| TI TMS320DM355 ZCE IBIS MODEL
[IBIS ver] 3.2
[File_name] sprm271a.ibs
[File Rev]   1.30
[Date]   October 24, 2007
[Source]   TIH DSP design
[Notes]   This data is based on 3/14/06 package substrate.
   Voltage of IO is VDDS +5%, -10%.
   EM_A08/10/11 are changed from PD to PU. [1.10]
   Updated pin file   [1.20]
   Updated some of IO model   [1.20]
   ADDED DDR pins support   [1.30]
[Disclaimer]   This information is for modeling purpose only, and is
   not guaranteed.
   The information is subject to change without notice.
[Copyright]   Property of Texas Instruments Incorporated. Unauthorized
   reproduction and/or distribution is strictly prohibited. This
   product is protected under copyright law and trade secret law
   as an unpublished work. Copyright (C) 2006, Texas Instruments
   Incorporated, all rights reserved. These commodities are under
   the U.S. Government distribution license control. As such,
   they are not to be re-exported without the prior approval of
   the U.S. Department of Commerce.
| Component   TMS320DM355 ZCE
[Component]   TMS320DM355ZCE
[Manufacturer] Texas Instruments
[Package]
| variable   typ   min   max
R_pkg   2.34767E-001  1.09280E-001  3.31800E-001
L_pkg   3.54436E-009  1.69380E-009  6.02860E-009
C_pkg   7.29148E-013  4.32190E-013  1.42590E-012
[Pin]signal_name   model_name   R_pin   L_pin   C_pin
G3   EXTCLK   BC3325DTHYPD   2.24E-01   3.68E-09   6.78E-13
C3   YOUT7   BC3325DTHYPD   1.96E-01   3.10E-09   4.95E-13
B3   YOUT4   BC3325DTHYPD   2.78E-01   4.88E-09   7.97E-13
B4   YOUT5   BC3325DTHYPD   3.26E-01   6.03E-09   9.32E-13
A4   YOUT6   BC3325DTHYPD   2.71E-01   4.71E-09   7.32E-13
B2   YOUT3   BC3325DTHYPD   2.52E-01   4.56E-09   8.47E-13
A3   YOUT2   BC3325DTHYPD   2.98E-01   5.52E-09   8.15E-13
A2   YOUT1   BC3325DTHYPD   2.79E-01   5.46E-09   8.87E-13
B1   YOUT0   BC3325DTHYPD   2.68E-01   4.80E-09   8.71E-13
D2   COUT6   BC3325DTHYPD   2.51E-01   3.93E-09   7.90E-13
L5   YIN7   BC3350CTHYPD   1.39E-01   2.19E-09   7.55E-13
N3   CIN7   BC3350CTHYPD   2.40E-01   3.18E-09   9.57E-13
M3   CIN5   BC3350CTHYPD   2.64E-01   3.86E-09   7.08E-13
M4   YIN6   BC3350CTHYPD   2.64E-01   3.41E-09   1.04E-12
P5   YIN0   BC3350CTHYPD   2.60E-01   3.76E-09   1.22E-12
M5   YIN5   BC3350CTHYPD   2.98E-01   4.46E-09   1.34E-12
R3   YIN3   BC3350CTHYPD   2.77E-01   4.03E-09   8.58E-13
P4   YIN2   BC3350CTHYPD   2.01E-01   2.55E-09   8.40E-13
P3   YIN4   BC3350CTHYPD   2.67E-01   3.81E-09   9.00E-13
P2   YIN1   BC3350CTHYPD   2.97E-01   4.54E-09   1.18E-12
H5   LCD_OE   BC3325DTHYPD   2.32E-01   3.10E-09   6.60E-13
H4   FIELD   BC3325DTHYPD   1.86E-01   2.46E-09   5.37E-13
G5   VSYNC   BC3325DTHYPD   1.82E-01   2.38E-09   5.53E-13
F5   HSYNC   BC3325DTHYPD   2.28E-01   3.17E-09   7.08E-13
J9   VSSA_PLL2   GND   NA   NA   NA
H12   VSSA_PLL1   GND   NA   NA   NA
R11   VSSA_DLL   GND   NA   NA   NA
U10   VREFSSTL   POWER   NA   NA   NA
R10   VDDAHV33_DLL   POWER   NA   NA   NA
H9   VDDA_PLL2   POWER   NA   NA   NA
E8   EMU0   BC3325DTHYPU   2.57E-01   3.30E-09   1.02E-12
G12   VDDA_PLL1   POWER   NA   NA   NA
D11   RESETN   IC33THYPU   2.56E-01   3.26E-09   8.09E-13
C11   CLKOUT3   BC3350CTHYPD   1.96E-01   2.57E-09   7.51E-13
H3   VCLK   BC3325DSHYPD   1.87E-01   2.45E-09   5.52E-13
R17   UART1_TXD   BC3350ASHYPD   1.86E-01   2.72E-09   6.26E-13
R15   UART1_RXD   BC3350ASHYPD   2.02E-01   2.70E-09   9.58E-13
U18   UART0_RXD   IC33SHYPD   2.32E-01   3.57E-09   7.82E-13
T18   UART0_TXD   OC3350AS   2.16E-01   3.33E-09   6.87E-13
D8   TMS   IC33THYPU   2.63E-01   3.30E-09   7.20E-13
D9   TDI   IC33THYPU   2.81E-01   3.50E-09   6.13E-13
E9   TDO   OC3325DT   2.44E-01   2.99E-09   7.89E-13
E10   TCK   IC33THYPU   3.10E-01   4.93E-09   8.89E-13
E12   SPI1_SDO   BC3350CTHYPD   2.02E-01   2.75E-09   6.28E-13
A13   SPI1_SDI   BC3350CTHYPD   2.58E-01   4.15E-09   5.96E-13
C13   SPI1_SCLK   BC3350CTHYPD   2.04E-01   2.76E-09   7.60E-13
E13   SPI1_SDENA0   BC3350CTHYPD   2.79E-01   3.93E-09   8.91E-13
D14   MMCSD0_DATA1   BC3350CTHYPD   2.61E-01   3.43E-09   8.23E-13
B11   SPI0_SDO   BC3350CTHYPD   2.51E-01   3.72E-09   6.74E-13
D12   CLKOUT1   BC3350CTHYPD   2.25E-01   3.01E-09   6.78E-13
A12   SPI0_SDI   BC3350CTHYPD   2.34E-01   3.88E-09   6.07E-13
B12   SPI0_SDENA0   BC3350CTHYPD   2.70E-01   3.75E-09   6.15E-13
C12   SPI0_SCLK   BC3350CTHYPD   2.21E-01   3.17E-09   6.93E-13
E14   GIO001   BC3365ATHYPD   2.35E-01   3.09E-09   1.05E-12
J3   CIN0   BC3350CTHYPD   2.70E-01   4.04E-09   8.54E-13
B16   MMCSD1_DATA3   BC3350CTHYPD   2.33E-01   3.81E-09   6.66E-13
A15   MMCSD0_CLK   BC3350CTHYPD   2.67E-01   4.46E-09   6.01E-13
C16   GIO000   BC3365ATHYPD   2.73E-01   4.09E-09   8.36E-13
A16   MMCSD1_DATA2   BC3350CTHYPD   2.48E-01   4.17E-09   5.81E-13
B15   MMCSD1_DATA1   BC3350CTHYPD   2.44E-01   3.74E-09   6.10E-13
A17   MMCSD1_CMD   BC3350CTHYPD   2.74E-01   4.58E-09   6.24E-13
A18   MMCSD1_DATA0   BC3350CTHYPD   2.77E-01   5.82E-09   7.92E-13
C14   MMCSD0_CMD   BC3350CTHYPD   2.27E-01   3.65E-09   7.84E-13
C15   MMCSD1_CLK   BC3350CTHYPD   2.06E-01   2.68E-09   7.39E-13
B18   GIO006   BC3365ATHYPD   2.87E-01   4.64E-09   6.99E-13
A14   MMCSD0_DATA3   BC3350CTHYPD   2.62E-01   4.19E-09   5.94E-13
B13   MMCSD0_DATA2   BC3350CTHYPD   2.56E-01   3.91E-09   6.43E-13
B14   MMCSD0_DATA0   BC3350CTHYPD   2.30E-01   3.51E-09   9.89E-13
E11   RTCK   OC3325DT   2.48E-01   3.31E-09   6.96E-13
C9   TRSTN   IC33THYPD   2.04E-01   2.63E-09   4.65E-13
T3   PCLK   BC3350CTHYPD   1.22E-01   2.38E-09   8.68E-13
E16   ASP1_FSX   BC3350BSHYPD   1.82E-01   2.59E-09   1.05E-12
F17   ASP0_CLKR   BC3350BSHYPD   2.24E-01   2.88E-09   7.42E-13
D17   ASP1_CLKS   IC33SHYPD   2.03E-01   3.10E-09   8.02E-13
E17   ASP1_FSR   BC3350BSHYPD   2.46E-01   3.84E-09   7.20E-13
F16   ASP0_FSR   BC3350BSHYPD   1.79E-01   2.30E-09   8.28E-13
D19   ASP1_CLKX   BC3350BSHYPD   2.53E-01   4.18E-09   5.69E-13
C18   ASP1_DX   BC3350BSHYPD   2.24E-01   3.75E-09   6.87E-13
D18   ASP1_CLKR   BC3350BSHYPD   2.11E-01   3.33E-09   5.56E-13
C19   ASP1_DR   BC3350BSHYPD   2.56E-01   4.43E-09   6.92E-13
G17   ASP0_FSX   BC3350BSHYPD   1.71E-01   2.28E-09   5.88E-13
E18   ASP0_DR   BC3350BSHYPD   2.30E-01   3.86E-09   6.62E-13
H15   ASP0_DX   BC3350BSHYPD   1.79E-01   2.34E-09   6.24E-13
G19   EM_CE1   BC3350CSHYPD   2.40E-01   4.05E-09   5.45E-13
F18   ASP0_CLKX   BC3350BSHYPD   2.16E-01   3.38E-09   6.61E-13
R13   I2C_SDA   BC3350BSHYPD   3.22E-01   4.17E-09   1.13E-12
R14   I2C_SCL   BC3350BSHYPD   2.43E-01   3.14E-09   1.02E-12
E4   COUT2   BC3325DTHYPD   2.20E-01   3.31E-09   6.32E-13
C17   GIO007   BC3350CTHYPD   2.25E-01   3.48E-09   7.55E-13
D15   GIO005   BC3365ATHYPD   2.11E-01   2.63E-09   8.41E-13
B17   GIO004   BC3365ATHYPD   2.72E-01   4.04E-09   6.65E-13
G15   GIO003   BC3365ATHYPD   2.63E-01   3.75E-09   1.12E-12
F15   GIO002   BC3365ATHYPD   3.18E-01   4.17E-09   1.13E-12
E7   EMU1   BC3325DTHYPU   2.77E-01   3.78E-09   9.43E-13
J15   EM_WE   BC3350CSHYPD   1.83E-01   2.47E-09   6.58E-13
H16   EM_ADV   BC3350CSHYPD   1.69E-01   2.18E-09   6.65E-13
F19   EM_OE   BC3350CSHYPD   2.53E-01   4.47E-09   6.15E-13
G18   EM_WAIT   BC3350CSHYPU   2.11E-01   3.12E-09   6.97E-13
E19   EM_CLK   BC3350CSHYPD   2.53E-01   4.48E-09   7.16E-13
H18   EM_D00   BC3350CSHYPD   2.09E-01   3.17E-09   5.66E-13
J16   EM_CE0   BC3350CSHYPD   1.88E-01   2.45E-09   7.90E-13
K18   EM_D09   BC3350CSHYPD   2.09E-01   3.14E-09   5.13E-13
L17   EM_D11   BC3350CSHYPD   1.70E-01   2.32E-09   6.00E-13
K19   EM_D07   BC3350CSHYPD   2.30E-01   3.76E-09   4.32E-13
L16   EM_D08   BC3350CSHYPD   1.80E-01   2.42E-09   5.40E-13
K17   EM_D06   BC3350CSHYPD   1.74E-01   2.35E-09   6.18E-13
L19   EM_D10   BC3350CSHYPD   2.30E-01   3.75E-09   4.84E-13
J19   EM_D05   BC3350CSHYPD   2.32E-01   3.80E-09   5.15E-13
J18   EM_D03   BC3350CSHYPD   2.09E-01   3.10E-09   5.35E-13
L15   EM_D04   BC3350CSHYPD   1.86E-01   2.61E-09   7.42E-13
H19   EM_D02   BC3350CSHYPD   2.33E-01   3.84E-09   5.25E-13
J17   EM_D01   BC3350CSHYPD   1.82E-01   2.38E-09   5.78E-13
M18   EM_D15   BC3350CSHYPD   2.01E-01   3.08E-09   7.29E-13
M19   EM_D14   BC3350CSHYPD   2.37E-01   3.99E-09   5.53E-13
M15   EM_D13   BC3350CSHYPD   1.88E-01   2.62E-09   6.90E-13
L18   EM_D12   BC3350CSHYPD   2.41E-01   3.76E-09   6.14E-13
P19   EM_BA1   BC3350CSHYPD   2.49E-01   4.15E-09   6.53E-13
N19   EM_BA0   BC3350CSHYPD   2.40E-01   4.22E-09   6.24E-13
M16   EM_A00   BC3350CSHYPD   1.96E-01   2.56E-09   8.14E-13
P17   EM_A09   BC3350CSHYPD   1.71E-01   2.45E-09   6.27E-13
R18   EM_A10   BC3350CSHYPU   2.32E-01   3.69E-09   6.83E-13
T19   EM_A08   BC3350CSHYPU   2.60E-01   4.63E-09   7.18E-13
P18   EM_A06   BC3350CSHYPD   2.26E-01   3.53E-09   7.06E-13
P16   EM_A07   BC3350CSHYPD   1.77E-01   2.36E-09   9.18E-13
P15   EM_A04   BC3350CSHYPD   1.87E-01   2.60E-09   9.81E-13
R19   EM_A05   BC3350CSHYPD   2.54E-01   4.40E-09   7.09E-13
N18   EM_A03   BC3350CSHYPD   2.21E-01   3.25E-09   6.71E-13
N15   EM_A02   BC3350CSHYPD   1.83E-01   2.49E-09   9.24E-13
N17   EM_A01   BC3350CSHYPD   2.28E-01   3.20E-09   7.44E-13
V19   EM_A13   BC3350CSHYPD   2.56E-01   4.94E-09   6.57E-13
U19   EM_A12   BC3350CSHYPD   2.70E-01   4.79E-09   6.54E-13
R16   EM_A11   BC3350CSHYPU   1.84E-01   2.61E-09   7.83E-13
C2   COUT7   BC3325DTHYPD   2.66E-01   4.58E-09   8.29E-13
D3   COUT4   BC3325DTHYPD   2.14E-01   3.45E-09   7.31E-13
C1   COUT5   BC3325DTHYPD   2.56E-01   4.23E-09   7.11E-13
E3   COUT3   BC3325DTHYPD   2.71E-01   4.04E-09   8.99E-13
F3   COUT1   BC3325DTHYPD   3.20E-01   5.25E-09   1.12E-12
F4   COUT0   BC3325DTHYPD   1.79E-01   2.48E-09   5.17E-13
A11   CLKOUT2   BC3350CTHYPD   2.34E-01   3.76E-09   5.69E-13
K5   CIN6   BC3350CTHYPD   2.85E-01   4.98E-09   1.14E-12
L4   CIN4   BC3350CTHYPD   1.30E-01   1.89E-09   5.85E-13
J4   CIN3   BC3350CTHYPD   2.78E-01   4.31E-09   9.42E-13
L3   CIN1   BC3350CTHYPD   2.57E-01   3.51E-09   7.66E-13
J5   CIN2   BC3350CTHYPD   2.52E-01   4.09E-09   9.26E-13
R5   CAM_WEN_FIELD   BC3350CTHYPD   2.80E-01   3.85E-09   1.03E-12
N5   CAM_HD   BC3350CTHYPD   3.32E-01   4.97E-09   1.43E-12
R4   CAM_VD   BC3350CTHYPD   2.67E-01   3.52E-09   9.37E-13
T8   DDR_CS   BCSSTL18TCSCGPBFZP33   2.60E-01   3.33E-09   9.15E-13
V12   DDR_DQS0   BCSSTL18TCSCGPBFZP33   2.28E-01   3.17E-09   5.83E-13
V15   DDR_DQS1   BCSSTL18TCSCGPBFZP33   2.47E-01   3.53E-09   5.24E-13
W15   DDR_DQ11   BCSSTL18TCSCGPBFZP33   2.65E-01   3.98E-09   4.84E-13
W16   DDR_DQ13   BCSSTL18TCSCGPBFZP33   2.71E-01   4.35E-09   5.28E-13
U11   DDR_DQ2   BCSSTL18TCSCGPBFZP33   2.31E-01   3.04E-09   6.83E-13
V11   DDR_DQ0   BCSSTL18TCSCGPBFZP33   2.29E-01   3.12E-09   6.24E-13
U15   DDR_DQM1   BCSSTL18TCSCGPBFZP33   1.95E-01   2.57E-09   6.49E-13
W14   DDR_DQ10   BCSSTL18TCSCGPBFZP33   2.38E-01   3.67E-09   6.26E-13
V14   DDR_DQ9   BCSSTL18TCSCGPBFZP33   2.12E-01   3.09E-09   6.33E-13
U13   DDR_DQ8   BCSSTL18TCSCGPBFZP33   2.55E-01   3.13E-09   7.02E-13
V13   DDR_DQ6   BCSSTL18TCSCGPBFZP33   2.09E-01   3.15E-09   6.82E-13
W13   DDR_DQ7   BCSSTL18TCSCGPBFZP33   2.63E-01   3.96E-09   6.05E-13
U12   DDR_DQ4   BCSSTL18TCSCGPBFZP33   2.32E-01   3.04E-09   6.87E-13
W12   DDR_DQ5   BCSSTL18TCSCGPBFZP33   2.34E-01   4.00E-09   6.69E-13
T11   DDR_DQ3   BCSSTL18TCSCGPBFZP33   1.09E-01   1.69E-09   7.03E-13
W11   DDR_DQ1   BCSSTL18TCSCGPBFZP33   2.52E-01   3.71E-09   5.81E-13
U16   DDR_DQ12   BCSSTL18TCSCGPBFZP33   2.10E-01   3.07E-09   7.26E-13
V9   DDR_CAS   BCSSTL18TCSCGPBFZP33   2.28E-01   3.16E-09   6.48E-13
W9   DDR_CLKP   BCSSTL18TCSCGPBFZP33   2.28E-01   3.32E-09   6.12E-13
W8   DDR_CLKN   BCSSTL18TCSCGPBFZP33   2.27E-01   3.47E-09   5.96E-13
U6   DDR_A13   BCSSTL18TCSCGPBFZP33   1.93E-01   2.59E-09   7.80E-13
V10   DDR_CKE   BCSSTL18TCSCGPBFZP33   2.11E-01   3.10E-09   6.55E-13
V8   DDR_BA2   BCSSTL18TCSCGPBFZP33   2.04E-01   3.00E-09   6.39E-13
U8   DDR_BA0   BCSSTL18TCSCGPBFZP33   2.45E-01   3.10E-09   7.55E-13
U7   DDR_BA1   BCSSTL18TCSCGPBFZP33   2.22E-01   2.98E-09   6.50E-13
W6   DDR_A9   BCSSTL18TCSCGPBFZP33   2.62E-01   4.13E-09   5.43E-13
W7   DDR_A11   BCSSTL18TCSCGPBFZP33   2.55E-01   4.01E-09   5.72E-13
V5   DDR_A7   BCSSTL18TCSCGPBFZP33   2.15E-01   3.31E-09   5.94E-13
W5   DDR_A8   BCSSTL18TCSCGPBFZP33   2.62E-01   4.00E-09   5.05E-13
V6   DDR_A10   BCSSTL18TCSCGPBFZP33   2.09E-01   3.14E-09   6.17E-13
U5   DDR_A6   BCSSTL18TCSCGPBFZP33   1.95E-01   2.56E-09   7.42E-13
W4   DDR_A5   BCSSTL18TCSCGPBFZP33   2.67E-01   4.23E-09   5.04E-13
V4   DDR_A4   BCSSTL18TCSCGPBFZP33   2.23E-01   3.46E-09   6.09E-13
W3   DDR_A3   BCSSTL18TCSCGPBFZP33   2.78E-01   4.36E-09   5.80E-13
W2   DDR_A2   BCSSTL18TCSCGPBFZP33   2.83E-01   4.51E-09   6.46E-13
V3   DDR_A1   BCSSTL18TCSCGPBFZP33   2.34E-01   3.38E-09   6.40E-13
V7   DDR_A12   BCSSTL18TCSCGPBFZP33   2.05E-01   3.13E-09   6.01E-13
V2   DDR_A0   BCSSTL18TCSCGPBFZP33   2.79E-01   4.39E-09   7.45E-13
V17   DDR_STRBEN_DEL   BCSSTL18TCSCGPBFZP33   2.41E-01   3.55E-09   6.91E-13
W18   DDR_STRBEN   BCSSTL18TCSCGPBFZP33   2.97E-01   4.73E-09   6.68E-13
V16   DDR_DQ14   BCSSTL18TCSCGPBFZP33   2.61E-01   3.71E-09   6.02E-13
T6   DDR_RAS   BCSSTL18TCSCGPBFZP33   2.24E-01   3.24E-09   1.02E-12
W10   DDR_WE   BCSSTL18TCSCGPBFZP33   2.45E-01   3.86E-09   6.36E-13
T12   DDR_DQM0   BCSSTL18TCSCGPBFZP33   1.95E-01   2.53E-09   7.28E-13
W17   DDR_DQ15   BCSSTL18TCSCGPBFZP33   2.59E-01   4.27E-09   6.01E-13
|   Model Selecter
[Model Selector] BC3325DTHYPU
BC3325DSHYPU_3.3_PUZ  Cell operated at 3.3(nom) PULLUP_OFF
BC3325DSHYPU_3.3_PU  Cell operated at 3.3(nom) PULLUP_ON
[Model Selector] BC3325DSHYPU
BC3325DSHYPU_3.3_PUZ  Cell operated at 3.3(nom) PULLUP_OFF
BC3325DSHYPU_3.3_PU  Cell operated at 3.3(nom) PULLUP_ON
[Model Selector] OC3325DT
BC3325DSHYPD_3.3_PDZ  Cell operated at 3.3(nom) PULLDOWN_OFF
[Model Selector] BC3325DSHYPD
BC3325DSHYPD_3.3_PDZ  Cell operated at 3.3(nom) PULLDOWN_OFF
BC3325DSHYPD_3.3_PD  Cell operated at 3.3(nom) PULLDOWN_ON
[Model Selector] BC3325DTHYPD
BC3325DSHYPD_3.3_PDZ  Cell operated at 3.3(nom) PULLDOWN_OFF
BC3325DSHYPD_3.3_PD  Cell operated at 3.3(nom) PULLDOWN_ON
[Model Selector] OC3350AS
BC3350ASHYPD_3.3_PDZ  Cell operated at 3.3(nom) PULLDOWN_OFF
[Model Selector] BC3350ASHYPD
BC3350ASHYPD_3.3_PDZ  Cell operated at 3.3(nom) PULLDOWN_OFF
BC3350ASHYPD_3.3_PD  Cell operated at 3.3(nom) PULLDOWN_ON
[Model Selector] BC3350BSHYPD
BC3350BSHYPD_PDZ_3P3  Cell operated at 3.3(nom) PULLDOWN_OFF
BC3350BSHYPD_PD_3P3  Cell operated at 3.3(nom) PULLDOWN_ON
[Model Selector] BC3350CTHYPD
BC3350CSHYPD_3.3_PDZ  Cell operated at 3.3(nom) PULLDOWN_OFF
BC3350CSHYPD_3.3_PD  Cell operated at 3.3(nom) PULLDOWN_ON |
[Model Selector] BC3350CSHYPD
BC3350CSHYPD_3.3_PDZ  Cell operated at 3.3(nom) PULLDOWN_OFF
BC3350CSHYPD_3.3_PD  Cell operated at 3.3(nom) PULLDOWN_ON
[Model Selector] BC3350CSHYPU
BC3350CSHYPU_3.3_PUZ  Cell operated at 3.3(nom) PULLUP_OFF
BC3350CSHYPU_3.3_PU  Cell operated at 3.3(nom) PULLUP_ON
[Model Selector] BC3365ATHYPD
BC3365ATHYPD_3.3_PDZ  Cell operated at 3.3(nom) PULLDOWN_OFF
BC3365ATHYPD_3.3_PD  Cell operated at 3.3(nom) PULLDOWN_ON
[Model Selector] BCSSTL18TCSCGPBFZP33
MOS_NO_SR0_FULL_TERM  Cell operated at 1.8(nom) CMOS_NO_SR0_FULL_TERM
SSTL_NO_SR0_NO_TERM  Cell operated at 1.8(nom) SSTL_NO_SR0_NO_TERM
STL_NO_SR0_FULL_TERM  Cell operated at 1.8(nom) SSTL_NO_SR0_FULL_TERM
MOS_NO_SR0_HALF_TERM  Cell operated at 1.8(nom) CMOS_NO_SR0_HALF_TERM
STL_NO_SR0_HALF_TERM  Cell operated at 1.8(nom) SSTL_NO_SR0_HALF_TERM
CMOS_NO_SR0_NO_TERM  Cell operated at 1.8(nom) CMOS_NO_SR0_NO_TERM
NO_SR0_NO_TERM  Cell operated at 1.8(nom) NO_SR0
SR0_NO_TERM  Cell operated at 1.8(nom) SR0
[Model Selector] IC33SHYPD
IC33THYPD_PDZ   PULDOWN_OFF
IC33THYPD_PD   PULLDOWN_ON
[Model Selector] IC33THYPD
IC33THYPD_PDZ   PULDOWN_OFF
IC33THYPD_PD   PULLDOWN_ON
[Model Selector] IC33THYPU
IC33THYPU_PUZ   PULLUP_OFF
IC33THYPU_PU   PULLUP_ON
| Models and submodels in the file (26): BC3325DSHYPD_3.3_PD (I/O), BC3325DSHYPD_3.3_PDZ (I/O), BC3325DSHYPU_3.3_PU (I/O), BC3325DSHYPU_3.3_PUZ (I/O), BC3350ASHYPD_3.3_PD (I/O), BC3350ASHYPD_3.3_PDZ (I/O), BC3350BSHYPD_PD_3P3 (I/O), BC3350BSHYPD_PDZ_3P3 (I/O), BC3350CSHYPD_3.3_PD (I/O), BC3350CSHYPD_3.3_PDZ (I/O), BC3350CSHYPU_3.3_PU (I/O), BC3350CSHYPU_3.3_PUZ (I/O), BC3365ATHYPD_3.3_PDZ (I/O), BC3365ATHYPD_3.3_PD (I/O), MOS_NO_SR0_FULL_TERM (Input), SSTL_NO_SR0_NO_TERM (Input), STL_NO_SR0_FULL_TERM (Input), MOS_NO_SR0_HALF_TERM (Input), STL_NO_SR0_HALF_TERM (Input), CMOS_NO_SR0_NO_TERM (Input), NO_SR0_NO_TERM (I/O), SR0_NO_TERM (I/O), IC33THYPD_PDZ (Input), IC33THYPD_PD (Input), IC33THYPU_PUZ (Input), IC33THYPU_PU (Input)
